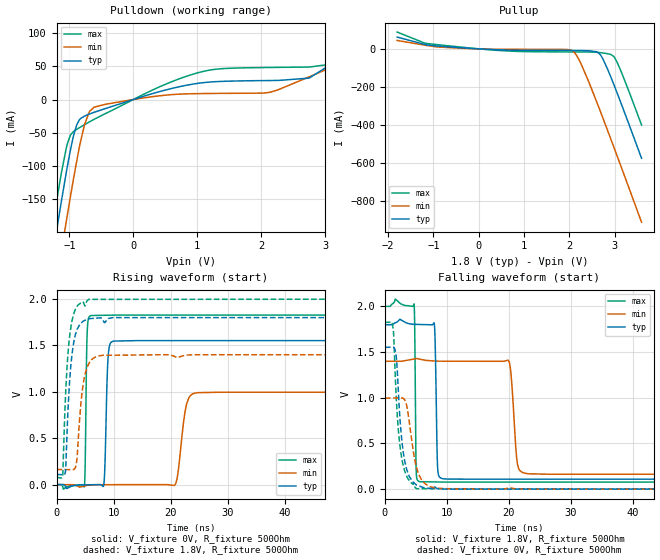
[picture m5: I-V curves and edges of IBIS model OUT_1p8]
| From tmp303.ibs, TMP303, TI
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|   Model
[Model]   OUT_1p8
Model_type   Output
Polarity   Non-Inverting
Vmeas = 0.9
Vref = 0
Cref = 1pF
Rref = 100000
|   typ   min   max
C_comp   1pF   1pF   1pF
[Voltage Range]   1.8   1.4   2
[Temperature Range]   25   125   -40
[Pullup Reference]   1.8   1.4   2
[Pulldown Reference]   -0   -0   -0
[Power Clamp Reference]   1.8   1.4   2
[GND Clamp Reference]   -0   -0   -0
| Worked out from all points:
|   slope of the pulldown table from 0 to 0.27 V, typ, clamps not added: 33.3 ohm
|   slope of the pullup table from 0 to 0.27 V, typ, clamps not added: 80.8 ohm
|   falling waveform, V_fixture 1.8V, R_fixture 500Ohm: 20-80 % time 252ps typ, 691ps min, 150ps max; typ from 1.8 V to 0.109 V
|   rising waveform, V_fixture 0V, R_fixture 500Ohm: 20-80 % time 394ps typ, 1.12ns min, 231ps max; typ from 0 V to 1.55 V
|   rising waveform, V_fixture 1.8V, R_fixture 500Ohm: 20-80 % time 1.05ns typ, 1.14ns min, 1.05ns max; typ from 0.109 V to 1.8 V
|   falling waveform, V_fixture 0V, R_fixture 500Ohm: 20-80 % time 1.15ns typ, 1.47ns min, 1.11ns max; typ from 1.55 V to 0 V
[Pulldown]
|   Voltage   I(typ)   I(min)   I(max)
-1.8V     -578.7mA   -655.6mA   -533.3mA
-1.26V    -235.6mA   -313.1mA   -190.2mA
-1.174V   -183.1mA   -260mA     -138.9mA
-1.049V   -111.2mA   -185.4mA   -74.32mA
-882mV    -37.77mA   -91.81mA   -44.88mA
-757.8mV  -24.81mA   -36.47mA   -37.76mA
-612mV    -19.29mA   -11.55mA   -29.85mA
1.062V    25.17mA    8.995mA    41.81mA
2.12V     28.72mA    10.76mA    48.49mA
2.747V    32.35mA    34.22mA    49.12mA
3.049V    50.85mA    46.94mA    52.93mA
3.595V    87.67mA    69.14mA    108.7mA
[Pullup]
|   Voltage   I(typ)   I(min)   I(max)
-1.8V     61.79mA    44.13mA    88.07mA
-1.12V    19.74mA    16.54mA    27.35mA
532.8mV   -5.783mA   -2.307mA   -9.815mA
1.894V    -8.563mA   -3.06mA    -16.21mA
2.088V    -8.675mA   -14.11mA   -16.39mA
2.174V    -8.724mA   -40.03mA   -16.46mA
2.266V    -8.814mA   -82.44mA   -16.53mA
2.666V    -25.33mA   -316.3mA   -19.46mA
2.741V    -53.06mA   -363.5mA   -21.81mA
2.979V    -185.1mA   -513.8mA   -39.53mA
3.163V    -298.6mA   -631.4mA   -129.8mA
3.595V    -574.8mA   -910.9mA   -400mA
[Ramp]
R_load = 500
|   typ   min   max
dV/dt_r   0.931264/3.93816e-10   0.597767/1.12322e-09   1.09629/2.30891e-10
dV/dt_f   1.01454/2.51815e-10   0.742321/6.90848e-10   1.15359/1.50007e-10
[Falling Waveform]
V_fixture = 1.8V
V_fixture_min = 1.4V
V_fixture_max = 2V
R_fixture = 500Ohm
C_fixture = 0F
|   Time   V(typ)   V(min)   V(max)
0s        1.8V       1.4V       2V
4.707ns   1.804V     1.425V     2.021V
5.026ns   1.804V     1.429V     226.4mV
5.54ns    1.803V     1.424V     82.5mV
7.953ns   1.814V     1.404V     78.82mV
8.481ns   251.3mV    1.401V     78.26mV
9.225ns   115mV      1.401V     77.48mV
19.99ns   109.2mV    1.402V     77.41mV
22.83ns   109.2mV    170.9mV    77.41mV
100ns     109.1mV    162.8mV    77.34mV
[Rising Waveform]
V_fixture = 0V
V_fixture_min = 0V
V_fixture_max = 0V
R_fixture = 500Ohm
C_fixture = 0F
|   Time   V(typ)   V(min)   V(max)
0s        512.3pV    1.994nV    354.3pV
4.879ns   -3.063mV   -14.92mV   -19.27mV
5.376ns   -2.457mV   -7.589mV   1.644V
5.95ns    -1.758mV   -5.408mV   1.821V
8.255ns   -12.49mV   -1.108mV   1.825V
9.036ns   1.37V      -1.014mV   1.826V
9.846ns   1.545V     -916.3uV   1.827V
20.66ns   1.552V     -9.556mV   1.827V
24.29ns   1.552V     986.5mV    1.827V
100ns     1.552V     996.3mV    1.827V
[Rising Waveform]
V_fixture = 1.8V
V_fixture_min = 1.4V
V_fixture_max = 2V
R_fixture = 500Ohm
C_fixture = 0F
|   Time   V(typ)   V(min)   V(max)
0s        109.1mV    162.8mV    77.34mV
1.099ns   106.7mV    162.3mV    100.6mV
1.562ns   137.3mV    162.1mV    931.7mV
2.088ns   895.8mV    161.8mV    1.468V
2.638ns   1.361V     161.6mV    1.743V
3.46ns    1.646V     214.8mV    1.905V
4.576ns   1.756V     1.041V     1.972V
5.617ns   1.786V     1.297V     1.997V
8.128ns   1.775V     1.394V     1.997V
100ns     1.8V       1.4V       2V
[Falling Waveform]
|Gnd
V_fixture = 0V
V_fixture_min = 0V
V_fixture_max = 0V
R_fixture = 500Ohm
C_fixture = 0F
|   Time   V(typ)   V(min)   V(max)
0s        1.552V     996.3mV    1.827V
1.31ns    1.555V     997.8mV    1.762V
1.763ns   1.478V     998.3mV    1.084V
1.993ns   1.287V     998.5mV    801.7mV
2.747ns   518.3mV    999.4mV    321.6mV
3.46ns    227.7mV    927.1mV    150mV
5.103ns   44.81mV    233.8mV    4.751mV
6.609ns   13mV       52.3mV     4.675mV
10.32ns   78.89uV    2.8mV      4.489mV
100ns     512.3pV    1.987nV    354.3pV
